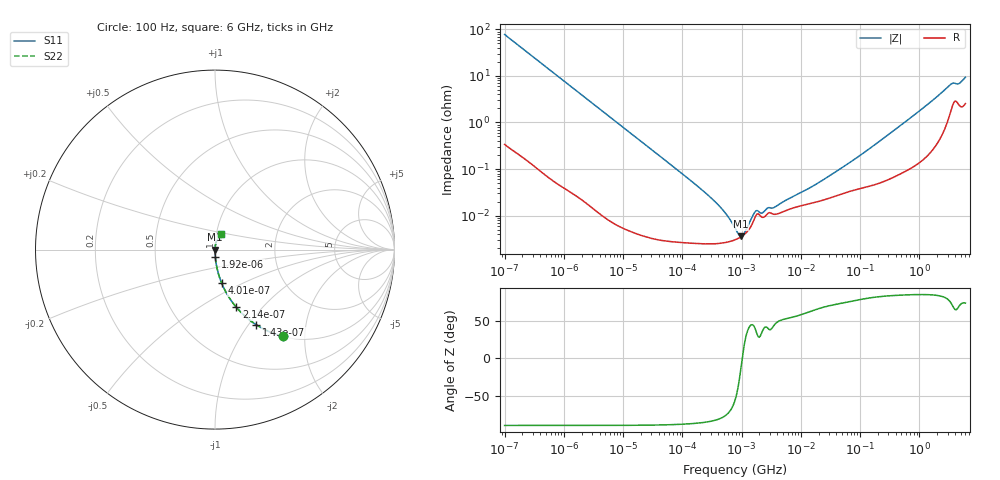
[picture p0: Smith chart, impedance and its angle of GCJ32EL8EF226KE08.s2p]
!Murata Part Number: GCJ32EL8EF226KE08
!These Parameters are Measured in Series Mode Connection
!Data Generated on Mar 13, 2026
!  o--ll--o
!Port1  Port2
!  o------o
!Operation Temp=25[degC], DC Bias Voltage=0[V]
!Freq. Start=100[Hz] Stop=6[GHz] 401[Steps]
# Hz S RI R 50
!Freq.(Hz) S11(Real) S11(Imag) S21(Real) S21(Imag) S12(Real) S12(Imag) S22(Real) S22(Imag)
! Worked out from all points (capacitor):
!   401 points, 100 Hz to 6 GHz, reference 50 ohm
!   read as one part in series: C = 20.4 uF near 109 Hz
!   lowest |Z| = 3.58 mohm at 969 kHz (marker M1)
!   series resonance near 1.025 MHz, so ESL is about 1.2 nH
!   S11 on the Smith chart (normalised r, x): 100 Hz: 1.01, -1.56; 143 Hz: 1.00, -1.09; 214 Hz: 1.00, -0.73; 401 Hz: 1.00, -0.39; 1.92 kHz: 1.00, -0.08; 6 GHz: 1.05, +0.18
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100  0.3781 -0.4828  0.6219 0.4828  0.6219 0.4828  0.3781 -0.4828
143  0.23 -0.4186  0.77 0.4186  0.77 0.4186  0.23 -0.4186
214  0.1185 -0.3209  0.8815 0.3209  0.8815 0.3209  0.1185 -0.3209
401  0.0375 -0.1877  0.9625 0.1877  0.9625 0.1877  0.0375 -0.1877
820  0.00949 -0.0946  0.9905 0.0946  0.9905 0.0946  0.00949 -0.0946
1920  0.0019 -0.0408  0.9981 0.0408  0.9981 0.0408  0.0019 -0.0408
2008  0.00174 -0.0391  0.9983 0.0391  0.9983 0.0391  0.00174 -0.0391
40335  3.37e-05 -0.00196  1 0.00196  1 0.00196  3.37e-05 -0.00196
241822  2.47e-05 -0.000311  1 0.000311  1 0.000311  2.47e-05 -0.000311
566185  2.67e-05 -9.87e-05  1 9.87e-05  1 9.87e-05  2.67e-05 -9.87e-05
774597  3.01e-05 -4.49e-05  1 4.49e-05  1 4.49e-05  3.01e-05 -4.49e-05
968953  3.46e-05 -9e-06  1 9e-06  1 9e-06  3.46e-05 -9e-06
1449809  5.94e-05 5.93e-05  0.9999 -5.93e-05  0.9999 -5.93e-05  5.94e-05 5.93e-05
1813585  0.000107 7e-05  0.9999 -7e-05  0.9999 -7e-05  0.000107 7e-05
2268635  9.12e-05 6.94e-05  0.9999 -6.94e-05  0.9999 -6.94e-05  9.12e-05 6.94e-05
2713602  0.000108 9.48e-05  0.9999 -9.48e-05  0.9999 -9.48e-05  0.000108 9.48e-05
1.555665e7  0.000185 0.000377  0.9998 -0.000377  0.9998 -0.000377  0.000185 0.000377
7.797396e7  0.000351 0.00153  0.9996 -0.00153  0.9996 -0.00153  0.000351 0.00153
3.124326e8  0.000635 0.00566  0.9994 -0.00566  0.9994 -0.00566  0.000635 0.00566
3.352442e9  0.0199 0.0608  0.9801 -0.0608  0.9801 -0.0608  0.0199 0.0608
4.586474e9  0.0276 0.06  0.9724 -0.06  0.9724 -0.06  0.0276 0.06
6e9  0.0323 0.085  0.9677 -0.085  0.9677 -0.085  0.0323 0.085
